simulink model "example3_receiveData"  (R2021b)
settings: Solver=FixedStepDiscrete  StartTime=0.0  StopTime=inf  FixedStep=0.1  RelTol=1e-3
undefined symbols (not defined in the file or in its folder): Endian, Little
libraries: CANBusLib x5, simulink x1

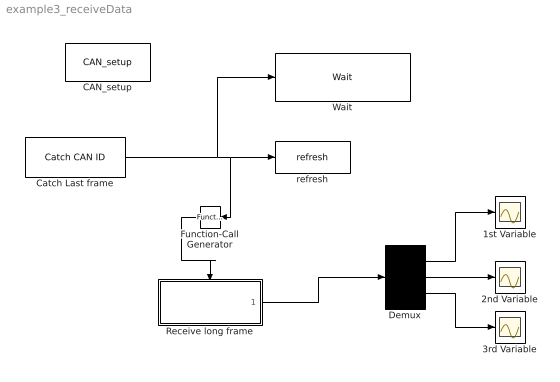
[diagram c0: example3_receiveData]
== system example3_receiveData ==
  1st Variable : Scope
  2nd Variable : Scope
  3rd Variable : Scope
  CAN_setup : CANBusLib/CAN_setup  Priority=1  g1_cmbPortName="\"COM17\""  g2_cmbBaudRate=250000  g3_chkEcho=off  g59_chkTerminator=on  g4_cmbObjectID=0  g5_chkEnableSync=off  g10_chkRxWDEnable=off  g12_cmbRxWDLen=1  g13_cmbRxWDStartPos=1  g_60_cmbRxWDMode=0  g15_chkTxWDEnable=off  g17_cmbTxWDLen=1  g18_cmbTxWDStartPos=1  g_61_cmbTxWDMode=0  g20_ediF1=0  g21_chkExt4F1=off  g22_ediF2=0  g23_chkExt4F2=off  g24_ediF3=0  g25_chkExt4F3=off  g26_ediF4=0  g27_chkExt4F4=off  g28_ediF5=0  g29_chkExt4F5=off  g30_ediF6=0  g31_chkExt4F6=off  g32_ediF7=0  g33_chkExt4F7=off  g34_ediF8=0  g35_chkExt4F8=off  g36_ediM1=0  g37_ediF9=0  g38_chkExt4F9=on  g39_ediF10=0  g40_chkExt4F10=on  g41_ediF11=0  g42_chkExt4F11=on  g43_ediF12=0  g44_chkExt4F12=on  g45_ediM2=0  g46_ediF13=0  g47_chkExt4F13=off  g48_ediF14=0  g49_chkExt4F14=on  g50_ediF15=0  g51_chkExt4F15=on  g52_ediF16=0  g53_chkExt4F16=on  g54_ediM3=0  g62_autoFresh=off
  Catch Last frame : CANBusLib/Catch CAN ID  Priority=1  g1_ObjectID=0  g2_CANID=555  g3_Extended=off  g4_chkCatchLast=on  g5_lastFrameNo=1
  Demux : Demux  Priority=1  Outputs=3
  Function-Call Generator : simulink/Ports & Subsystems/Function-Call Generator  sample_time=1  numberOfIterations=1  DisallowWideOutput=off  ShowEnablePort=on
  Receive long frame : Subsystem  Priority=1  TreatAsAtomicUnit=on
  Wait : CANBusLib/Wait  Waitms=300
  refresh : CANBusLib/refresh  g1_cmbObjectID=0
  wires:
  Demux/1 -> 1st Variable/1
  Demux/2 -> 2nd Variable/1
  Demux/3 -> 3rd Variable/1
  Receive long frame/1(Out1) -> Demux/1
  Catch Last frame/1 -> Wait/1, refresh/1, Function-Call Generator/1
  Function-Call Generator/1 -> Receive long frame/Trigger

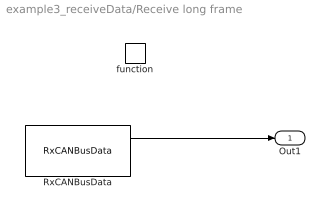
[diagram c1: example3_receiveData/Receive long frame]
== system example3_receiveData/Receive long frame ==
  function : TriggerPort  TriggerType=function-call  VariantControl=(inherit)
  RxCANBusData : CANBusLib/RxCANBusData  Priority=1  g1_ObjectID=0  g2_CANID=555  g3_Extended=off  g4_Datatype="\"int32\""  g5_Endian=Little-Endian  g6_Longframe=on  g7_OutDataQTY=3  g8_FirstFrameNo=0
  Out1 : Outport
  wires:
  RxCANBusData/1 -> Out1/1
